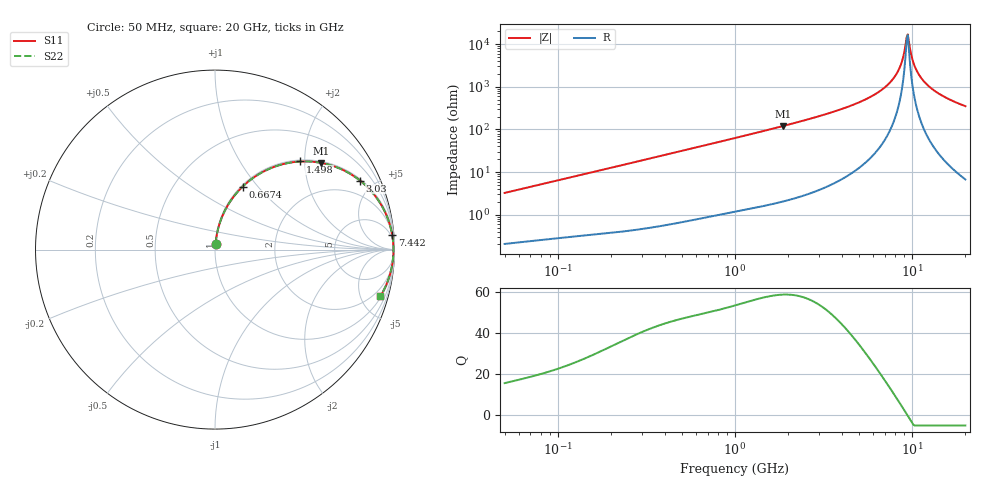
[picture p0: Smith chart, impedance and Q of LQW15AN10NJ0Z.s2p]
!Murata Part Number: LQW15AN10NJ0Z
!These Parameters are Measured in Series Mode Connection
!  o--[Z]--o
!Port1  Port2
!  o-------o
!Freq. Start=50[MHz] Stop=20[GHz], 401[Steps]
# Hz S RI R 50
!Freq.(Hz) S11(Real) S11(Imag) S21(Real) S21(Imag) S12(Real) S12(Imag) S22(Real) S22(Imag)
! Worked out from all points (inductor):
!   401 points, 50 MHz to 20 GHz, reference 50 ohm
!   read as one part in series: L = 10.2 nH near 51.52 MHz
!   highest Q = 59 at 1.876 GHz (marker M1), where L = 10.2 nH
!   self-resonance near 9.317 GHz
!   S11 on the Smith chart (normalised r, x): 50 MHz: 1.00, +0.06; 667.4 MHz: 1.02, +0.84; 1.498 GHz: 1.03, +1.90; 3.03 GHz: 1.08, +4.17; 7.442 GHz: 3, +24; 20 GHz: 1.13, -7.03
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5e7  0.00309 0.0322  0.9969 -0.0322  0.9969 -0.0322  0.00309 0.0322
1.364002e8  0.0105 0.0854  0.9895 -0.0854  0.9895 -0.0854  0.0105 0.0854
3.721004e8  0.0564 0.2196  0.9436 -0.2196  0.9436 -0.2196  0.0564 0.2196
6.673612e8  0.1541 0.3511  0.8459 -0.3511  0.8459 -0.3511  0.1541 0.3511
1e9  0.2868 0.4431  0.7132 -0.4431  0.7132 -0.4431  0.2868 0.4431
1.498439e9  0.4759 0.4908  0.5241 -0.4908  0.5241 -0.4908  0.4759 0.4908
1.875929e9  0.5919 0.4831  0.4081 -0.4831  0.4081 -0.4831  0.5919 0.4831
2.728004e9  0.7677 0.4134  0.2323 -0.4134  0.2323 -0.4134  0.7677 0.4134
3.029571e9  0.8087 0.3841  0.1913 -0.3841  0.1913 -0.3841  0.8087 0.3841
5.352748e9  0.9539 0.1943  0.0461 -0.1943  0.0461 -0.1943  0.9539 0.1943
6.503449e9  0.9775 0.1267  0.0225 -0.1267  0.0225 -0.1267  0.9775 0.1267
7.442007e9  0.9875 0.0803  0.0125 -0.0803  0.0125 -0.0803  0.9875 0.0803
8.389408e9  0.9926 0.0394  0.00737 -0.0394  0.00737 -0.0394  0.9926 0.0394
8.774992e9  0.9937 0.0241  0.00634 -0.0241  0.00634 -0.0241  0.9937 0.0241
9.178299e9  0.9942 0.00878  0.0058 -0.00878  0.0058 -0.00878  0.9942 0.00878
9.457416e9  0.9943 -0.00142  0.0057 0.00142  0.0057 0.00142  0.9943 -0.00142
9.600142e9  0.9943 -0.00652  0.00573 0.00652  0.00573 0.00652  0.9943 -0.00652
1.004137e10  0.9939 -0.0218  0.00614 0.0218  0.00614 0.0218  0.9939 -0.0218
1.034674e10  0.9933 -0.032  0.00667 0.032  0.00667 0.032  0.9933 -0.032
1.166392e10  0.989 -0.073  0.011 0.073  0.011 0.073  0.989 -0.073
1.460232e10  0.9712 -0.1506  0.0288 0.1506  0.0288 0.1506  0.9712 -0.1506
2e10  0.9208 -0.2606  0.0792 0.2606  0.0792 0.2606  0.9208 -0.2606
